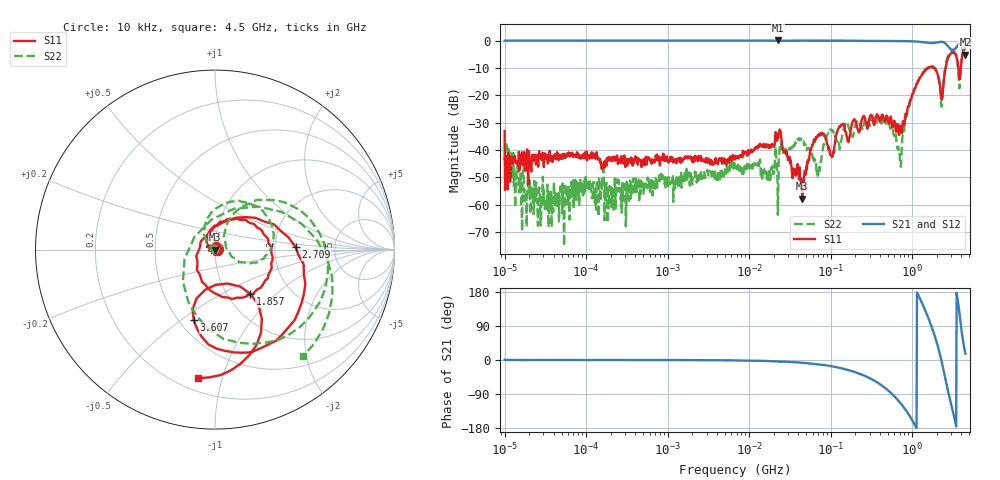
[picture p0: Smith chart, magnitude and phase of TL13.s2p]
!Siglent Technologies,SNA5004A,SNA5XCED5R0097,V1.0.0.2.10.R9
!Date: 2024-11-24 17:36:46
!Data & Calibration Information:
!Freq	S11:F2(ON)	S21:F2(ON)	S12:F2(ON)	S22:F2(ON)
# Hz S RI R 50
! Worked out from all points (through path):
!   1001 points, 10 kHz to 4.5 GHz, reference 50 ohm
!   highest |S21| = 0.10 dB at 22.8 MHz (marker M1); lowest = -5.0 dB at 4.5 GHz (marker M2)
!   group delay of S21, straight-line fit = 438 ps
!   lowest |S11| = -57.8 dB at 44.87 MHz (marker M3), VSWR 1.00, Z = 49.9 - j0.0938 ohm
!   |S11| at or under -10 dB: start of sweep to 1.573 GHz; 1.862 GHz to 2.569 GHz (707.3 MHz wide, 31.9 % of centre); 3.681 GHz to 3.949 GHz (268.5 MHz wide, 7.04 % of centre)
!   |S22| runs from -75.1 to -2.3 dB; largest |S21 - S12| = 0.02
!   S11 on the Smith chart (normalised r, x): 10 kHz: 1.00, +0.04; 1.857 GHz: 1.27, -0.70; 2.709 GHz: 2.63, +0.09; 3.607 GHz: 0.59, -0.56; 4.5 GHz: 0.28, -0.84
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10000  0.00293 0.0221  0.9999 0.0117  0.9977 0.0108  -0.00441 0.00471
10812.33  0.00375 -0.00708  1.004 0.00041  1 0.000767  0.00445 0.00858
26893.3  0.00807 -0.000676  1.007 0.000722  1.001 -0.00104  0.000588 0.00182
87919.76  0.0071 0.000855  1.007 3.16e-05  1.001 -0.00241  0.00143 -0.00231
772988.4  0.00596 0.00219  1.006 -0.00199  1.001 -0.00442  0.00168 -0.00228
6708204  0.0027 0.0062  1.004 -0.019  0.9963 -0.0216  -0.00361 -0.00345
2.280385e7  -0.00937 0.0139  1.01 -0.0685  1.001 -0.0675  -0.0013 0.00154
4.487199e7  -0.000887 -0.00094  0.9983 -0.1287  0.9863 -0.1268  0.000878 0.0152
5.897837e7  0.0101 0.00595  0.9881 -0.1673  0.9802 -0.1666  -0.00452 0.0074
7.169534e7  0.00776 0.0182  0.9824 -0.2014  0.9742 -0.1995  0.000395 0.00445
9.546883e7  -0.000806 0.011  0.9662 -0.2658  0.9582 -0.2635  0.00711 0.019
2.313556e8  0.0223 0.0108  0.7956 -0.5981  0.7914 -0.5909  0.0119 0.0264
5.185364e8  0.0257 -0.0151  0.1369 -0.9788  0.1408 -0.9718  0.0278 0.0161
6.995248e8  -0.0131 -0.0166  -0.3451 -0.9223  -0.339 -0.9199  0.00191 0.00891
1.132327e9  0.0315 0.1556  -0.9664 -0.00804  -0.9617 -0.0135  -0.0508 0.153
1.856924e9  0.1976 -0.2483  0.3243 0.8508  0.3145 0.8471  0.3242 0.0488
2.286891e9  -0.0847 0.00955  0.9569 -0.0237  0.9494 -0.0143  0.0616 0.0105
2.708552e9  0.4495 0.0131  0.2166 -0.7838  0.2244 -0.7772  0.4324 0.242
3.085101e9  0.379 -0.4688  -0.4036 -0.554  -0.3928 -0.5592  0.6088 -0.2316
3.606682e9  -0.119 -0.3918  -0.7777 0.2517  -0.7766 0.2367  -0.0975 -0.3765
4.002521e9  0.2434 -0.3135  0.0891 0.7993  0.0698 0.7946  0.3709 0.2098
4.5e9  -0.0921 -0.7167  0.5364 0.1601  0.5313 0.1706  0.4917 -0.5936
